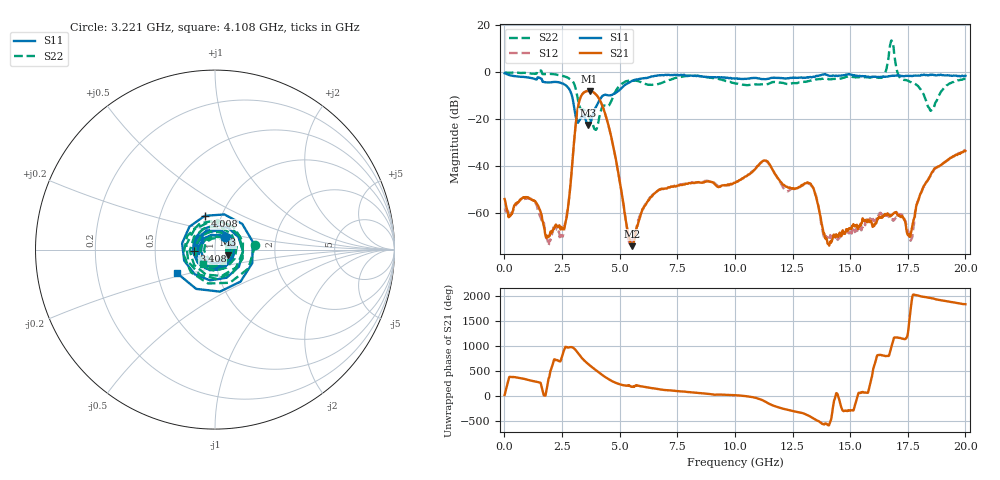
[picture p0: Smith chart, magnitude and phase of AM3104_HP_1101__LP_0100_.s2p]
!Created with skrf (http://scikit-rf.org).
# Hz S RI R 50.0
!freq ReS11 ImS11 ReS21 ImS21 ReS12 ImS12 ReS22 ImS22
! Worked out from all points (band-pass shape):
!   1601 points, 10 MHz to 20 GHz, reference 50 ohm
!   highest |S21| = -7.83 dB at 3.696 GHz (marker M1); lowest = -74.0 dB at 5.545 GHz (marker M2)
!   |S21| within 3 dB of the highest: 3.294 GHz to 4.089 GHz (794.6 MHz wide, 21.5 % of centre)
!   lowest |S11| = -22.3 dB at 3.621 GHz (marker M3), VSWR 1.17, Z = 57.5 - j3.34 ohm
!   |S11| at or under -10 dB: 2.934 GHz to 4.255 GHz (1.321 GHz wide, 36.7 % of centre)
!   |S22| runs from -24.4 to 13.6 dB; largest |S21 - S12| = 0.018
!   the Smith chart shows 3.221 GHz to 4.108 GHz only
!   S11 on the Smith chart (normalised r, x): 3.221 GHz: 1.11, +0.16; 3.408 GHz: 0.79, -0.02; 4.008 GHz: 0.83, +0.33; 4.108 GHz: 0.63, -0.18
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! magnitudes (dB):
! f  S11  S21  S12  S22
! 10 MHz  -0.4  -53.9  -57.9  -0.1
! 1.147 GHz  -2.3  -54.0  -53.9  -0.5
! 1.859 GHz  -4.3  -69.7  -71.2  -0.6
! 2.496 GHz  -4.6  -66.0  -69.4  -1.4
! 2.746 GHz  -6.2  -58.3  -57.7  -2.2
! 3.221 GHz  -20.9  -13.4  -13.5  -12.9
! 3.346 GHz  -19.2  -9.7  -9.8  -15.8
! 3.408 GHz  -18.4  -8.9  -9.0  -15.7
! 3.621 GHz  -22.3  -7.8  -7.9  -18.3
! 3.696 GHz  -22.1  -7.8  -7.9  -19.3
! 4.008 GHz  -14.1  -9.7  -9.8  -23.9
! 4.108 GHz  -12.1  -11.2  -11.2  -19.5
! 5.545 GHz  -3.6  -74.0  -71.4  -3.5
! 6.682 GHz  -1.2  -50.2  -50.2  -4.9
! 10.01 GHz  -2.7  -47.0  -47.1  -4.7
! 11.32 GHz  -2.9  -37.6  -37.9  -5.0
! 13.34 GHz  -2.0  -48.2  -48.4  -3.4
! 14.09 GHz  -1.5  -73.8  -70.0  -2.9
! 16.68 GHz  -1.6  -60.5  -61.6  7.1
! 17.64 GHz  -1.4  -68.3  -71.4  -4.2
! 18.5 GHz  -1.1  -43.5  -43.9  -16.3
! 20 GHz  -1.4  -33.4  -33.0  -2.7
